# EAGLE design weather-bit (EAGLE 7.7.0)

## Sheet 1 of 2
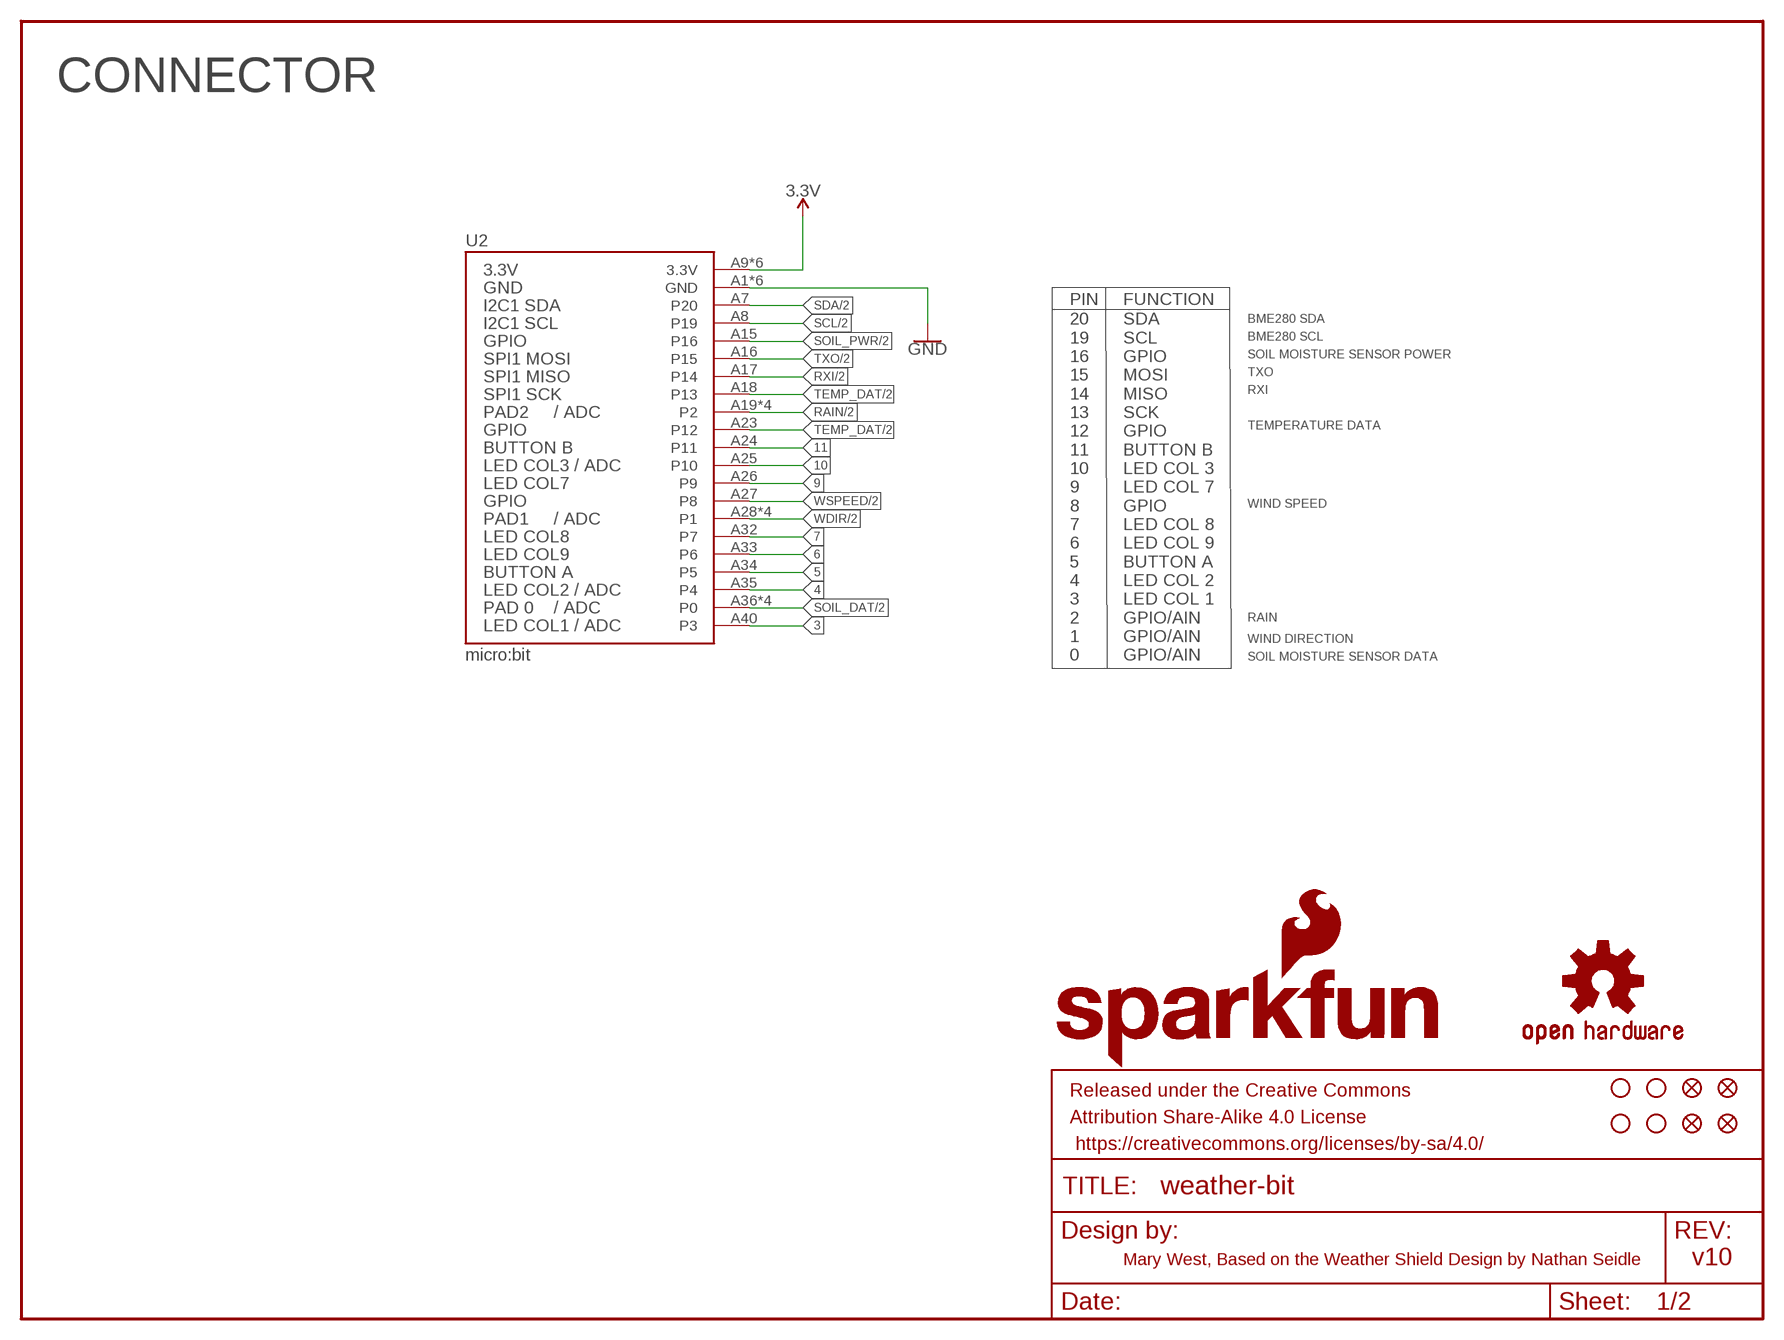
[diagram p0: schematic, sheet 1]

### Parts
FD1  FIDUCIAL1X2  [FIDUCIAL-1X2]
FD2  FIDUCIAL1X2  [FIDUCIAL-1X2]
FD3  FIDUCIAL1X2  [FIDUCIAL-1X2]
FD4  FIDUCIAL1X2  [FIDUCIAL-1X2]
FRAME1  FRAME-LETTER  [CREATIVE_COMMONS]
H1  STAND-OFF  [STAND-OFF]
H2  STAND-OFF  [STAND-OFF]
H3  STAND-OFF  [STAND-OFF]
H4  STAND-OFF  [STAND-OFF]
LOGO2  SFE_LOGO_NAME_FLAME.3_INCH  [SFE_LOGO_NAME_FLAME_.3]
LOGO3  OSHW-LOGOL  [OSHW-LOGO-L]
U2  micro:bit  MICRO:BITLEDS_UP  [MICRO:BIT_RA_PTH]

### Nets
3: U2.A40(P3)
3.3V: U2.A9(3.3V) U2.A10(3.3V) U2.A11(3.3V) U2.A12(3.3V) U2.A13(3.3V) U2.A14(3.3V) ; also sheet 2
4: U2.A35(P4)
5: U2.A34(P5)
6: U2.A33(P6)
7: U2.A32(P7)
9: U2.A26(P9)
10: U2.A25(P10)
11: U2.A24(P11)
GND: U2.A1(GND) U2.A2(GND) U2.A3(GND) U2.A4(GND) U2.A5(GND) U2.A6(GND) ; also sheet 2
RAIN: U2.A19(P2) U2.A20(P2) U2.A21(P2) U2.A22(P2) ; also sheet 2
RXI: U2.A17(P14) ; also sheet 2
SCL: U2.A8(P19) ; also sheet 2
SDA: U2.A7(P20) ; also sheet 2
SOIL_DAT: U2.A36(P0) U2.A37(P0) U2.A38(P0) U2.A39(P0) ; also sheet 2
SOIL_PWR: U2.A15(P16) ; also sheet 2
TEMP_DAT: U2.A18(P13) U2.A23(P12) ; also sheet 2
TXO: U2.A16(P15) ; also sheet 2
WDIR: U2.A28(P1) U2.A29(P1) U2.A30(P1) U2.A31(P1) ; also sheet 2
WSPEED: U2.A27(P8) ; also sheet 2

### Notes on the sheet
- CONNECTOR
- PIN | FUNCTION
- BME280 SDA
- BME280 SCL
- SOIL MOISTURE SENSOR POWER
- TXO
- RXI
- TEMPERATURE DATA
- WIND SPEED
- RAIN
- WIND DIRECTION
- 20
  19
  16
  15
  14
  13
  12
  11
  10
  9
  8
  7
  6
  5
  4
  3
  2
  1
  0
- SDA
  SCL
  GPIO
  MOSI
  MISO
  SCK
  GPIO
  BUTTON B
  LED COL 3
  LED COL 7
  GPIO
  LED COL 8
  LED COL 9
  BUTTON A
  LED COL 2
  LED COL 1
  GPIO/AIN
  GPIO/AIN
  GPIO/AIN
- SOIL MOISTURE SENSOR DATA
- Mary West, Based on the Weather Shield Design by Nathan Seidle | v10

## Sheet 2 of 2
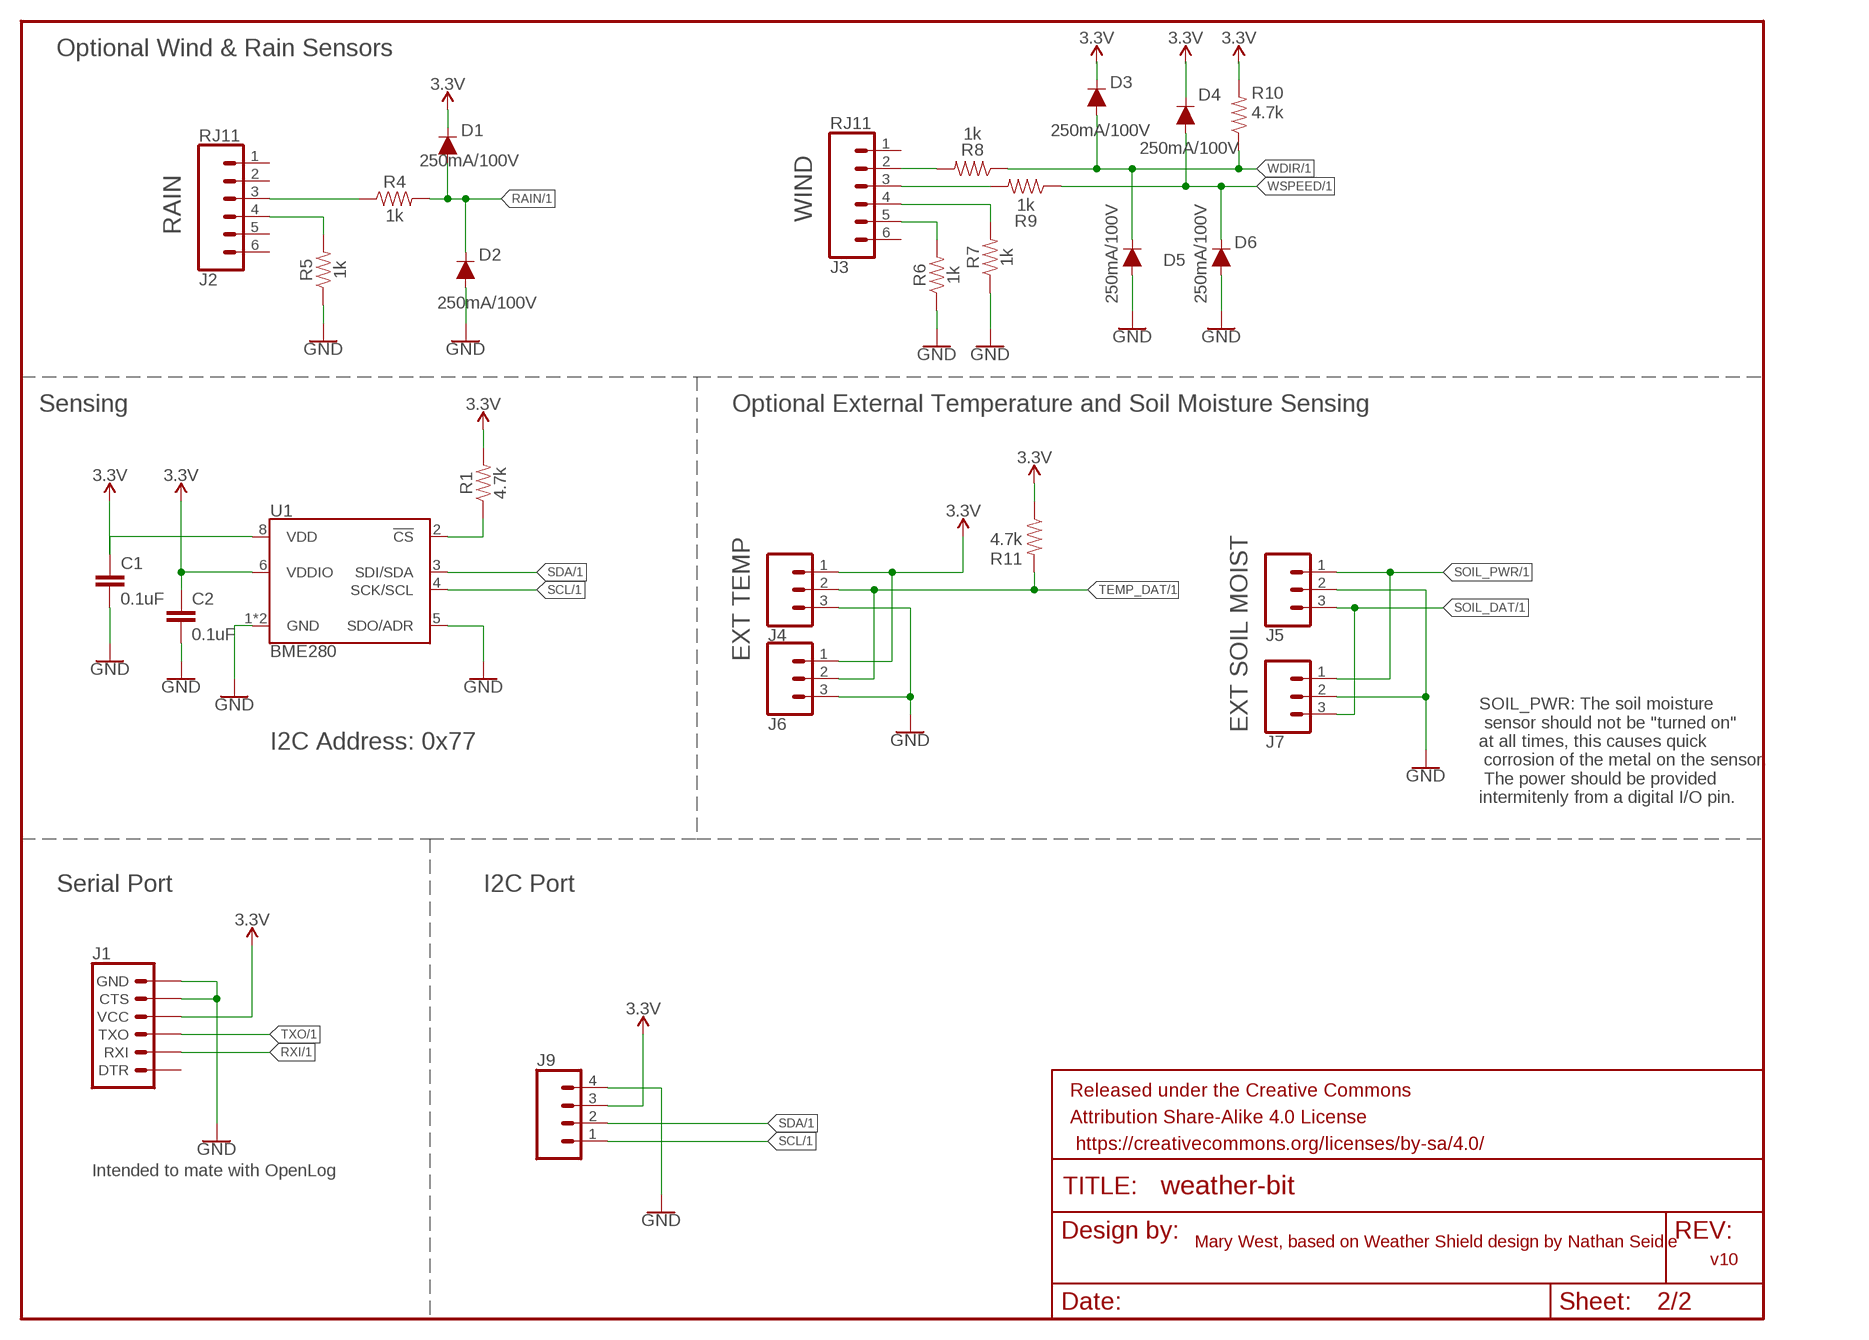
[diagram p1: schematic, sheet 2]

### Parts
C1  0.1uF  0.1UF-0603-25V-(+80/-20%)  [0603]
C2  0.1uF  0.1UF-0603-25V-(+80/-20%)  [0603]
D1  250mA/100V  DIODE-BAS16J  [SOD-323]
D2  250mA/100V  DIODE-BAS16J  [SOD-323]
D3  250mA/100V  DIODE-BAS16J  [SOD-323]
D4  250mA/100V  DIODE-BAS16J  [SOD-323]
D5  250mA/100V  DIODE-BAS16J  [SOD-323]
D6  250mA/100V  DIODE-BAS16J  [SOD-323]
FRAME2  FRAME-LETTER  [CREATIVE_COMMONS]
J1  6_PIN_SERIAL_TARGETSILK  [6_PIN_SERIAL_TARGET_SIDE_W_SILK]
J2  RJ11  RJ11-6  [RJ11-6]
J3  RJ11  RJ11-6  [RJ11-6]
J4  CONN_03SCREW_LOCK  [SCREWTERMINAL-3.5MM-3_LOCK.007S]
J5  CONN_03SCREW_LOCK  [SCREWTERMINAL-3.5MM-3_LOCK.007S]
J6  CONN_03  [1X03]
J7  CONN_03  [1X03]
J9  CONN_041X04_NO_SILK  [1X04_NO_SILK]
R1  4.7k  4.7KOHM-0603-1/10W-1%  [0603]
R4  1k  1KOHM-0603-1/10W-1%  [0603]
R5  1k  1KOHM-0603-1/10W-1%  [0603]
R6  1k  1KOHM-0603-1/10W-1%  [0603]
R7  1k  1KOHM-0603-1/10W-1%  [0603]
R8  1k  1KOHM-0603-1/10W-1%  [0603]
R9  1k  1KOHM-0603-1/10W-1%  [0603]
R10  4.7k  4.7KOHM-0603-1/10W-1%  [0603]
R11  4.7k  4.7KOHM-0603-1/10W-1%  [0603]
U1  BME280  [LGA-8-2.5X2.5]

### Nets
3.3V: C1.1 C2.1 D1.C D3.C D4.C J1.P$4(VCC) J4.1 J6.1 J9.3 R1.2 R10.2 R11.1 U1.6(VDDIO) U1.8(VDD) ; also sheet 1
GND: C1.2 C2.2 D2.A D5.A D6.A J1.P$5(CTS) J1.P$6(GND) J4.3 J5.2 J6.3 J7.2 J9.4 R5.1 R6.1 R7.1 U1.1(GND) U1.5(SDO/ADR) U1.7(GND) ; also sheet 1
N$2: R1.1 U1.2(!CS)
N$5: J2.3 R4.1
N$6: J3.2 R8.2
N$7: J2.4 R5.2
N$11: J3.3 R9.2
N$13: J3.5 R6.2
N$14: J3.4 R7.2
RAIN: D1.A D2.C R4.2 ; also sheet 1
RXI: J1.P$3(RXI) ; also sheet 1
SCL: J9.1 U1.4(SCK/SCL) ; also sheet 1
SDA: J9.2 U1.3(SDI/SDA) ; also sheet 1
SOIL_DAT: J5.3 J7.3 ; also sheet 1
SOIL_PWR: J5.1 J7.1 ; also sheet 1
TEMP_DAT: J4.2 J6.2 R11.2 ; also sheet 1
TXO: J1.P$2(TXO) ; also sheet 1
WDIR: D3.A D5.C R8.1 R10.1 ; also sheet 1
WSPEED: D4.A D6.C R9.1 ; also sheet 1
Unconnected: J1.P$1(DTR) J2.1 J2.2 J2.5 J2.6 J3.1 J3.6

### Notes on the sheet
- Optional Wind & Rain Sensors
- WIND
- RAIN
- Sensing | Optional External Temperature and Soil Moisture Sensing
- EXT TEMP
- EXT SOIL MOIST
- I2C Address: 0x77
- SOIL_PWR: The soil moisture
   sensor should not be "turned on" 
  at all times, this causes quick
   corrosion of the metal on the sensor.
   The power should be provided 
  intermitenly from a digital I/O pin.
- Serial Port | I2C Port
- Intended to mate with OpenLog
- Mary West, based on Weather Shield design by Nathan Seidle
- v10

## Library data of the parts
C1 C2 = SparkFun-Capacitors:0.1UF: 0.1µF ceramic capacitors; PROD_ID: CAP-00810
D1-D6 = SparkFun-DiscreteSemi:DIODE: Diode; PROD_ID: DIO-09646
FD1-FD4 = SparkFun-Aesthetics:FIDUCIAL: Fiducial Alignment Points
FRAME1 FRAME2 = SparkFun-Aesthetics:FRAME-LETTER: Schematic Frame - Letter
H1-H4 = SparkFun-Electromechanical:STAND-OFF: #4 Stand Off
J1 = SparkFun-Connectors:6_PIN_SERIAL_TARGET: 6-pin header connection for use with the "FTDI BASIC" pinout - TARGET SIDE. Also known as "Arduino Serial Program Header". It is used to mate with our FTDI Basic serial programmers using the Arduino IDE. Note, this device has "TARGET" in the name. It is intended to be used on a design that contains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
J2 J3 = SparkFun-Connectors:RJ11-6: RJ11 Jack - 6 pin Commonly found on CAT3 devices and some Microchip programmers. Here is the connector we sell at SparkFun: RJ11 6-Pin Connector (PRT-00132) Datasheet It is used on this SparkFun product: SparkFun Weather Shield (DEV-12081) Weather Meters (SEN-08942); PROD_ID: CONN-08590; SF_ID: PRT-00132
J4 J5 = SparkFun-Connectors:CONN_03: Multi connection point. Often used as Generic Header-pin footprint for 0.1 inch spaced/style header connections On any of the 0.1 inch spaced packages, you can populate with these: Break Away Headers - Straight (PRT-00116) Break Away Male Headers - Right Angle (PRT-00553) Female Headers (PRT-00115)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; PROD_ID: CONN-08288; SF_ID: PRT-08235
J6 J7 = SparkFun-Connectors:CONN_03: Multi connection point. Often used as Generic Header-pin footprint for 0.1 inch spaced/style header connections On any of the 0.1 inch spaced packages, you can populate with these: Break Away Headers - Straight (PRT-00116) Break Away Male Headers - Right Angle (PRT-00553) Female Headers (PRT-00115)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
J9 = SparkFun-Connectors:CONN_04: Multi connection point. Often used as Generic Header-pin footprint for 0.1 inch spaced/style header connections On any of the 0.1 inch spaced packages, you can populate with these: Break Away Headers - Straight (PRT-00116) Break Away Male Headers - Right Angle (PRT-00553) Female Headers (PRT-00115)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; PROD_ID: CONN-09696
LOGO2 = SparkFun-Aesthetics:SFE_LOGO_NAME_FLAME: SparkFun Font Logo w/ Flame
LOGO3 = SparkFun-Aesthetics:OSHW-LOGO: Open-Source Hardware (OSHW) Logo
R1 R10 R11 = SparkFun-Resistors:4.7KOHM: 4.7kΩ resistor; PROD_ID: RES-07857
R4-R9 = SparkFun-Resistors:1KOHM: 1kΩ resistor; PROD_ID: RES-07856
U1 = SparkFun-Sensors:BME280: Bosch BME280 &ndash; Combined Humidity and Pressure Sensor The BME280 is as combined digital humidity, pressure and temperature sensor based on proven sensing principles. The sensor module is housed in an extremely compact metal-lid LGA package with a footprint of only 2.5×2.5mm² with a height of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; PROD_ID: IC-13090
U2 = Micro_Bit_Parts:MICRO:BIT: BBC MICRO_BIT with 5x5 LED array facing the direction noted in the variant. "UP" means away from the host board, "Down" means facing towards the host board.; PROD_ID: CONN-13452

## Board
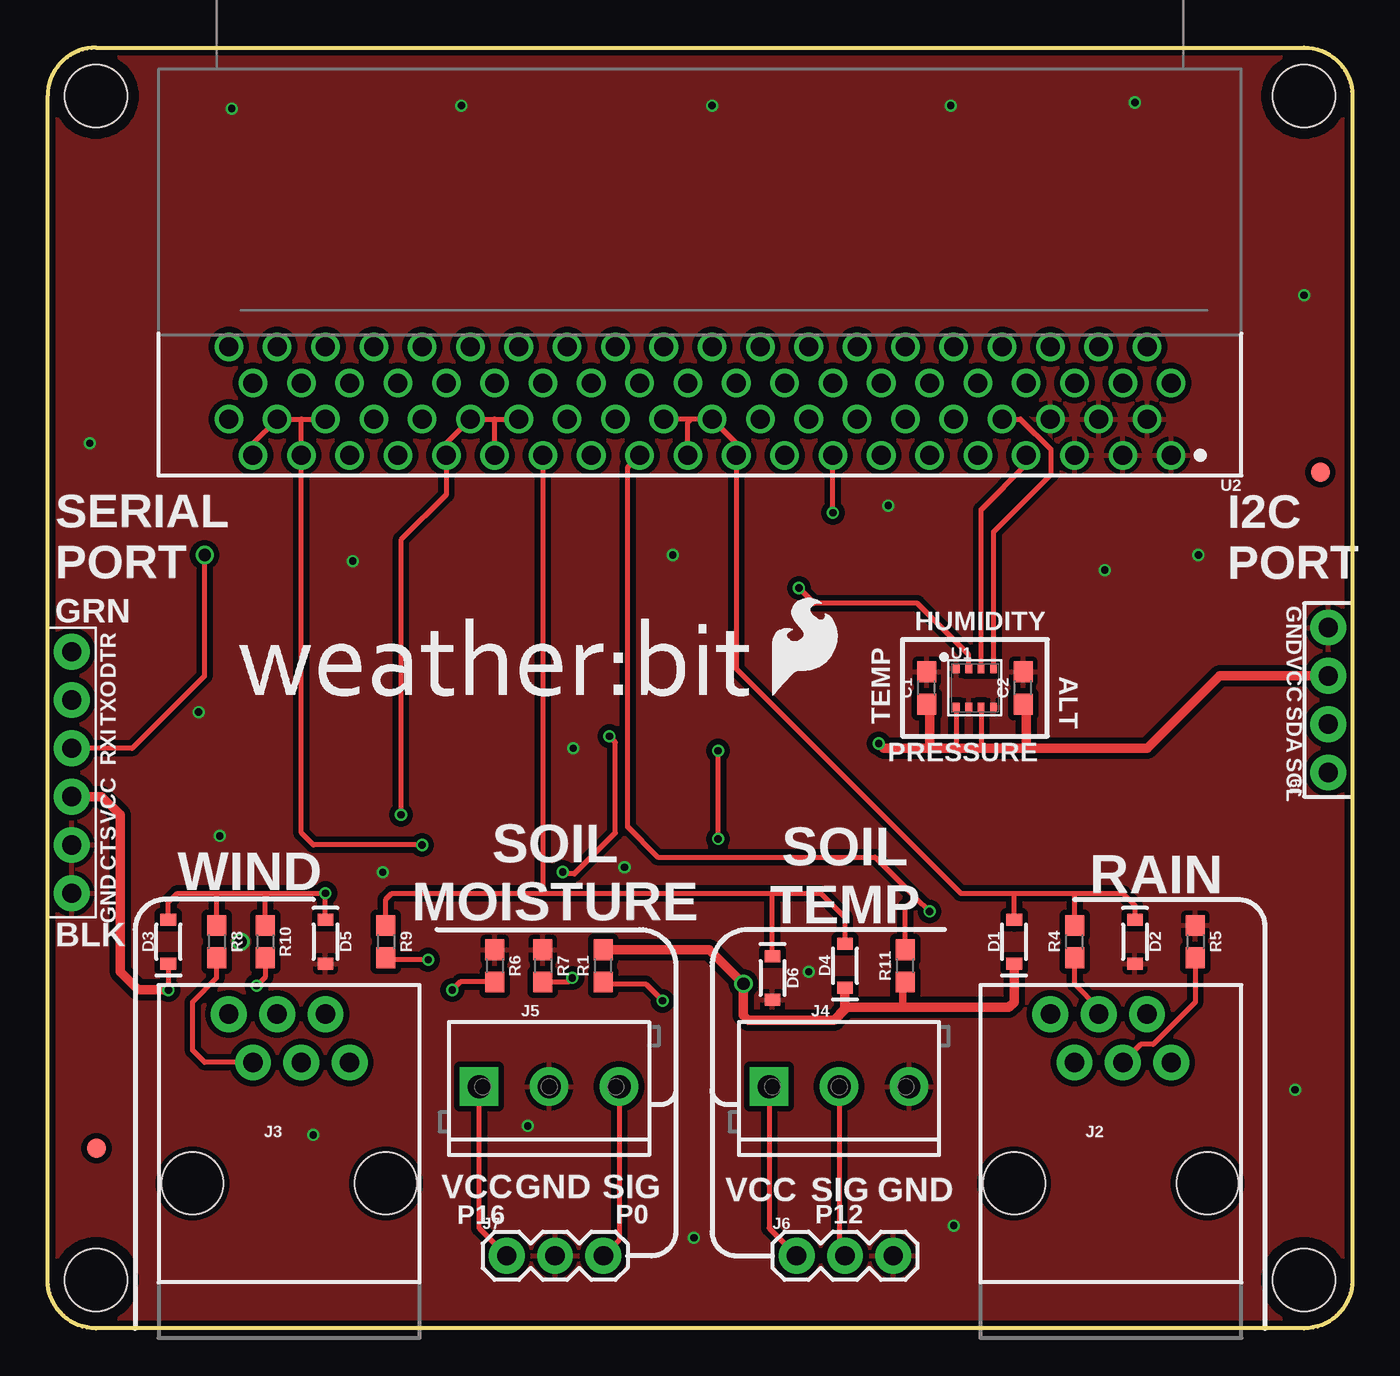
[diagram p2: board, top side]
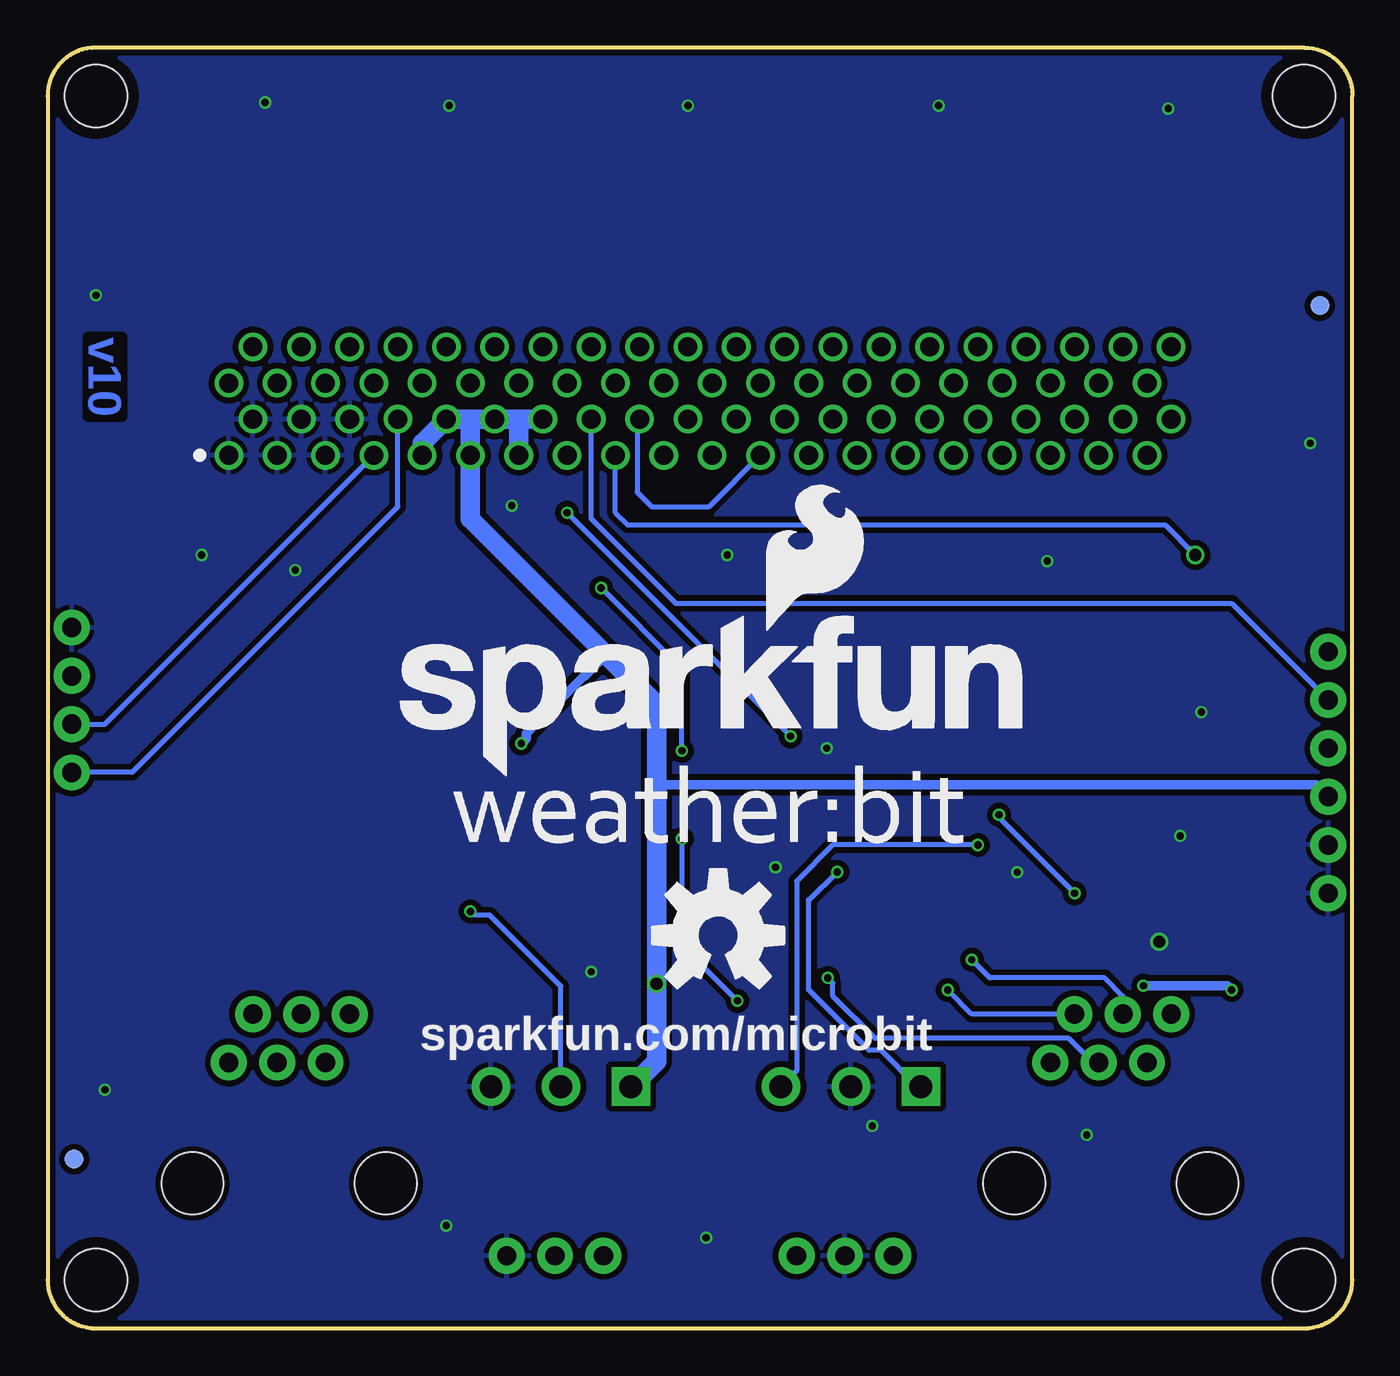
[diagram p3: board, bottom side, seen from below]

Size 68.58 x 67.31 mm. Coordinates in mm from the lower left corner, seen from the top.
Outline: 2.54,67.31 66.04,67.31 arc-90 68.58,64.77 68.58,2.54 arc-90 66.04,0 2.54,0 arc-90 0,2.54 0,64.77 arc-90 2.54,67.31
Copper layers (1*16): Top 0.035mm / dielectric 1.5mm / Bottom 0.035mm
Design rules "SparkFun-2-layer-FAB-LIMIT": minimum track width 4mil, minimum drill 6mil, track to track 4mil, track to pad 4mil, pad to pad 4mil, via to via 4mil, smd to smd 4mil, copper to edge 4mil, drill to drill 4mil, minimum pad ring 5mil, minimum via ring 5mil, stop-mask expansion 4mil, vias tented up to drill 25mil, thermal gap 10mil

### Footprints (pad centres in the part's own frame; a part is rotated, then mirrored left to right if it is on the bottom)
0603 = smd 1.1 x 1: 1 -0.85,0; 2 0.85,0
SOD-323 = smd 0.63 x 0.83: A 1.15,0; C -1.15,0
FIDUCIAL-1X2 = smd 1 x 1: 1 0,0
STAND-OFF = hole 3.302: 0,0
6_PIN_SERIAL_TARGET_SIDE_W_SILK = drill 1.016 pad 1.88: P$1 -6.35,0; P$2 -3.81,0; P$3 -1.27,0; P$4 1.27,0; P$5 3.81,0; P$6 6.35,0
RJ11-6 = drill 1.016 pad 1.88: 1 -3.175,8.89; 2 -1.905,6.35; 3 -0.635,8.89; 4 0.635,6.35; 5 1.905,8.89; 6 3.175,6.35 | hole 3.251: -5.08,0; 5.08,0
SCREWTERMINAL-3.5MM-3_LOCK.007S = drill 1.2 pad 2.032 square: 1 -0.178,0 | drill 1.2 pad 2.032: 2 3.5,0; 3 7.178,0
1X03 = drill 1.016 pad 1.88: 1 0,0; 2 2.54,0; 3 5.08,0
1X04_NO_SILK = drill 1.016 pad 1.88: 1 0,0; 2 2.54,0; 3 5.08,0; 4 7.62,0
LGA-8-2.5X2.5 = smd 0.35 x 0.5: 1 -0.975,1.025; 2 -0.325,1.025; 3 0.325,1.025; 4 0.975,1.025; 5 0.975,-1.025; 6 0.325,-1.025; 7 -0.325,-1.025; 8 -0.975,-1.025
MICRO:BIT_RA_PTH = drill 1: A1 -24.765,7.62; A2 -23.495,5.72; A3 -22.225,7.62; A4 -20.955,5.72; A5 -19.685,7.62; A6 -18.415,5.72; A7 -17.145,7.62; A8 -15.875,5.72; A9 -14.605,7.62; A10 -13.335,5.72; A11 -12.065,7.62; A12 -10.795,5.72; A13 -9.525,7.62; A14 -8.255,5.72; A15 -6.985,7.62; A16 -5.715,5.72; A17 -4.445,7.62; A18 -3.175,5.72; A19 -1.905,7.62; A20 -0.635,5.72; A21 0.635,7.62; A22 1.905,5.72; A23 3.175,7.62; A24 4.445,5.72; A25 5.715,7.62; A26 6.985,5.72; A27 8.255,7.62; A28 9.525,5.72; A29 10.795,7.62; A30 12.065,5.72; A31 13.335,7.62; A32 14.605,5.72; A33 15.875,7.62; A34 17.145,5.72; A35 18.415,7.62; A36 19.685,5.72; A37 20.955,7.62; A38 22.225,5.72; A39 23.495,7.62; A40 24.765,5.72; B1 -24.765,3.82; B2 -23.495,1.92; B3 -22.225,3.82; B4 -20.955,1.92; B5 -19.685,3.82; B6 -18.415,1.92; B7 -17.145,3.82; B8 -15.875,1.92; B9 -14.605,3.82; B10 -13.335,1.92; B11 -12.065,3.82; B12 -10.795,1.92; B13 -9.525,3.82; B14 -8.255,1.92; B15 -6.985,3.82; B16 -5.715,1.92; B17 -4.445,3.82; B18 -3.175,1.92; B19 -1.905,3.82; B20 -0.635,1.92; B21 0.635,3.82; B22 1.905,1.92; B23 3.175,3.82; B24 4.445,1.92; B25 5.715,3.82; B26 6.985,1.92; B27 8.255,3.82; B28 9.525,1.92; B29 10.795,3.82; B30 12.065,1.92; B31 13.335,3.82; B32 14.605,1.92; B33 15.875,3.82; B34 17.145,1.92; B35 18.415,3.82; B36 19.685,1.92; B37 20.955,3.82; B38 22.225,1.92; B39 23.495,3.82; B40 24.765,1.92

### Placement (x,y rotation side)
C1  46.2,33.66 90 top
C2  51.28,33.66 90 top
D1  50.8,20.32 90 top
D2  57.15,20.32 270 top
D3  6.35,20.32 90 top
D4  41.91,19.05 90 top
D5  14.61,20.32 270 top
D6  38.1,18.41 270 top
FD1  2.57,9.46 0 top
FD2  66.9,44.99 0 top
FD3  1.71,53.75 0 bottom
FD4  67.18,8.89 0 bottom
FRAME1  not placed on the board
FRAME2  not placed on the board
H1  2.54,64.77 0 top
H2  66.04,64.77 0 top
H3  2.54,2.54 0 top
H4  66.04,2.54 0 top
J1  1.27,29.21 270 top
J2  55.88,7.62 0 top
J3  12.7,7.62 0 top
J4  38.1,12.7 0 top
J5  22.86,12.7 0 top
J6  39.37,3.81 0 top
J7  24.13,3.81 0 top
J9  67.31,29.21 90 top
LOGO2  50.64,28.89 0 bottom
LOGO3  33.34,20.64 0 bottom
R1  29.21,19.05 90 top
R4  53.98,20.32 90 top
R5  60.33,20.32 270 top
R6  23.5,19.05 270 top
R7  26.04,19.05 270 top
R8  8.89,20.32 270 top
R9  17.78,20.32 270 top
R10  11.43,20.32 270 top
R11  45.09,19.05 90 top
U1  48.74,33.66 0 top
U2  34.29,53.5 180 top
U$1  [SFE_LOGO_FLAME_.2]  37.76,33.01 0 top
U$2  [LOGO-WEATHERBIT]  9.91,33.02 0 top
U$3  [LOGO-WEATHERBIT]  47.42,25.3 0 bottom
U$4  [ORDERING_INSTRUCTIONS]  not placed on the board

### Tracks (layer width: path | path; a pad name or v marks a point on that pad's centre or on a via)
3.3V  (via drill 0.38, 0.64)
  Top 0.254: J4.1 37.92,5.26 J6.1 | U1.8 47.76,30.62 47.62,30.48 | U1.6 49.06,30.65 48.9,30.48 | D3.C v6.35,17.78 | R10.2 11.43,18.45 v10.99,18 | 42.01,16.86 41.91,16.76
  Top 0.406: R11.1 44.96,18.2 44.96,16.86
  Top 0.508: 51.44,30.48 51.44,32.65 C2.1 | C1.1 46.35,32.65 46.35,30.48 | J9.3 61.59,34.29 57.78,30.48 51.44,30.48 | 51.44,30.48 48.9,30.48 47.62,30.48 46.35,30.48 | R1.2 34.77,19.9 v36.58,18.1 36.58,16.45 36.83,16.19 41.34,16.19 41.91,16.76 | J1.P$4 2.86,27.94 3.81,26.99 3.81,18.73 4.76,17.78 v6.35,17.78 | D1.C 50.8,17.14 50.51,16.86 44.96,16.86 42.01,16.86 41.91,16.95 D4.C | 46.35,30.48 43.94,30.48 v43.69,30.73
  Bottom 0.508: v10.99,18 6.57,18 v6.35,17.78 | 36.58,28.89 36.26,28.57 1.91,28.57 J1.P$4 | v43.69,30.73 43.43,30.99 43.43,31.24 40.39,34.29 40.32,34.29 39.21,35.4
  Bottom 1.016: U2.A14 43.81,47.78 | 43.81,47.78 U2.A12 46.2,47.78 | 46.2,47.78 U2.A10 48.9,46.51 U2.A9 | 46.2,47.78 46.35,47.62 U2.A11 46.35,42.55 39.21,35.4 36.58,32.77 36.58,28.89 v36.58,18.1 36.58,14.05 J4.1 | U2.A13 43.81,47.78
GND  (via drill 0.38, 0.64)
  other vias: 9.68,64.1 57.15,64.42 47.47,64.26 34.92,64.26 21.75,64.26 33.97,4.76 55.56,39.85 32.86,40.64 27.62,30.48 65.56,12.54 66.04,54.29 7.94,32.38 9.05,25.88 2.22,46.51 16.03,40.32 17.62,23.97 25.24,10.64 30.32,24.23 47.62,5.4 40.01,18.73 10.16,20.32 13.97,10.16 60.48,40.64 44.18,43.24
  pour Top (isolate 0.305): 0,67.31 -0.16,-0.32 68.42,-0.32 68.58,67.31
  pour Bottom (isolate 0.305): 0,67.31 -0.16,-0.32 68.42,-0.32 68.58,67.31
N$2  (via drill 0.38)
  Top 0.254: v35.24,25.72 v35.24,30.35 | R1.1 29.21,18.1 31.43,18.1 v32.32,17.21 | U1.2 48.41,35.41 45.72,38.1 40.3,38.1 v39.49,38.91
  Bottom 0.254: v35.24,30.35 35.24,34.66 v39.49,38.91 | v35.24,25.72 35.24,20.13 v32.32,17.21
N$5
  Top 0.254: J2.3 55.24,16.83 53.98,18.1 R4.1
N$6
  Top 0.254: J3.2 8.26,13.97 7.62,14.61 7.62,17.14 8.89,18.41 R8.2
N$7
  Top 0.254: R5.2 60.33,17.14 58.1,14.92 57.47,14.92 J2.4
N$11  (via drill 0.38)
  Top 0.254: v20,19.37 17.88,19.37 R9.2
  Bottom 0.254: J3.3 12.06,17.46 13.02,18.41 19.05,18.41 v20,19.37
N$13  (via drill 0.38)
  Top 0.254: R6.2 21.69,18.2 v21.27,17.78
  Bottom 0.254: J3.5 20,16.51 v21.27,17.78
N$14  (via drill 0.38)
  Top 0.254: R7.2 27.36,18.2 v27.57,18.41
  Bottom 0.254: J3.4 13.65,13.97 14.92,15.24 25.08,15.24 27.3,17.46 27.3,18.15 v27.57,18.41
RAIN
  Top 0.254: 50.8,21.27 D1.A 50.8,22.86 | 33.81,47.78 U2.A20 36.2,46.51 U2.A19 36.2,34.67 48.01,22.86 50.8,22.86 | 33.81,47.78 U2.A22 | U2.A21 33.66,47.62 33.81,47.78 | 50.8,22.86 53.98,22.86 | 53.98,22.86 56.52,22.86 57.15,22.23 D2.C | R4.2 53.98,22.86
RXI  (via drill 0.64)
  Top 0.254: J1.P$3 4.45,30.48 8.26,34.29 v8.26,40.64
  Bottom 0.254: U2.A17 38.73,42.86 38.1,42.23 9.84,42.23 v8.26,40.64
SCL
  Top 0.254: U2.A8 51.13,47.78 52.74,46.17 52.74,44.88 49.72,41.86 U1.4
  Bottom 0.254: U2.A8 50.16,43.18 64.14,29.21 J9.1
SDA
  Top 0.254: U2.A7 51.44,45.4 49.06,43.03 U1.3
  Bottom 0.254: J9.2 65.56,31.75 U2.A7
SOIL_DAT  (via drill 0.38)
  Top 0.254: J5.3 30.04,4.64 J7.3 | v19.68,25.4 13.97,25.4 13.34,26.04 U2.A37 13.34,47.78 | 13.34,47.78 U2.A38 10.79,46.51 U2.A39 | 13.34,47.78 U2.A36
  Bottom 0.254: v19.68,25.4 27.3,25.4 29.21,23.5 29.21,13.53 J5.3
SOIL_PWR  (via drill 0.38)
  Top 0.254: J7.1 22.68,5.26 J5.1 | v41.27,42.86 U2.A15 | v29.53,31.11 29.84,30.8 29.84,26.04 27.69,23.88 27.18,23.88 v27.08,23.98
  Bottom 0.254: v29.53,31.11 v41.27,42.86 | J5.1 22.86,12.7 24.77,14.61 25.4,14.61 28.57,17.78 28.57,22.54 28.51,22.54 v27.08,23.98
TEMP_DAT  (via drill 0.38)
  Top 0.254: J4.2 41.6,4.12 J6.2 | U2.A23 30.48,45.24 30.48,26.35 32.07,24.77 43.5,24.77 45.62,22.64 | 45.62,22.64 v46.35,21.91 | R11.2 45.09,22.1 45.62,22.64
  Bottom 0.254: U2.A18 37.59,47.78 37.59,43.94 36.83,43.18 33.81,43.18 U2.A23 | J4.2 41.6,17.98 45.34,21.72 46.16,21.72 v46.35,21.91
TXO
  Bottom 0.254: U2.A16 40.01,42.55 35.56,38.1 6.35,38.1 J1.P$2
WDIR  (via drill 0.38)
  Top 0.254: 23.5,47.78 U2.A30 20.95,46.51 U2.A31 20.95,43.81 18.57,41.43 v18.57,26.99 | 23.5,47.78 U2.A28 | U2.A29 23.5,47.78 | D3.A 6.35,22.38 6.83,22.86 8.89,22.86 | 8.89,22.86 11.59,22.86 | 11.59,22.86 v14.61,22.86 D5.C | R8.1 8.89,22.86 | R10.1 11.43,22.7 11.59,22.86
  Bottom 0.254: v18.57,26.99 18.57,26.83 v14.61,22.86
WSPEED
  Top 0.254: R9.1 17.78,22.54 18.1,22.86 26.19,22.86 | 26.19,22.86 38.1,22.86 | 38.1,22.86 40.64,22.86 41.91,21.59 D4.A | D6.C 38.1,22.86 | U2.A27 26.04,23.02 26.19,22.86

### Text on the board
Bottom: v10
tPlace: SERIAL / PORT | I2C / PORT | GND | HUMIDITY | VCC | ALT | SDA | TEMP | PRESSURE | SCL | SOIL / MOISTURE | SOIL / TEMP | WIND | RAIN | VCC | GND | SIG | VCC | SIG | GND | P0 | P12 | P16
bPlace: sparkfun.com/microbit
Measures: * All dimensions / are in inches
tDocu: Mary West, based on Weather Shield Design by Nathan Seidle | Solder Mask: Black Gloss

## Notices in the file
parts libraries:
SparkFun-Aesthetics: Licensing: Creative Commons ShareAlike 4.0 International - https://creativecommons.org/licenses/by-sa/4.0
SparkFun-Aesthetics: Released under the Creative Commons Attribution Share-Alike 4.0 License
SparkFun-Aesthetics: https://creativecommons.org/licenses/by-sa/4.0
